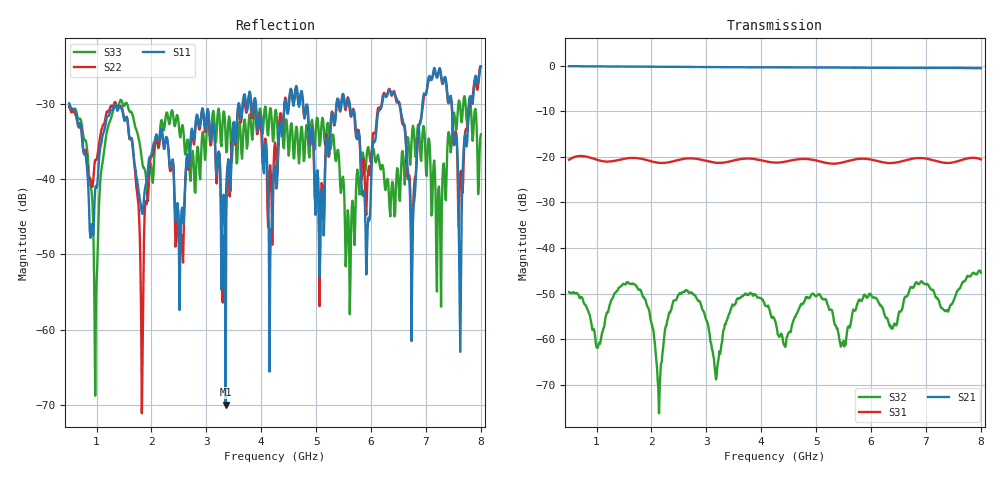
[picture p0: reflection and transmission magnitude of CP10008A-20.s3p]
! Amtery
! Email: info@amtery.com
! Phone: 886-2-2883-7839
! Model Number: CP10008A-20
! 3-port S-parameter measurement data for Directional Coupler
! Frequency Range: 0.5 GHz to 8 GHz
! Port 1: Input
! Port 2: Output
! Port 3: Coupled
# Hz S db R 50
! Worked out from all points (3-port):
!   601 points, 500 MHz to 8 GHz, reference 50 ohm
!   strongest paths, dB at 500 MHz, 2.375 GHz, 4.25 GHz, 6.125 GHz, 8 GHz:
!     S21: -0.1, -0.3, -0.4, -0.5, -0.6
!     S31: -20.6, -21.0, -21.3, -21.0, -20.6
!     S32: -49.7, -52.6, -55.9, -51.6, -45.4
!   lowest |S11| = -70.0 dB at 3.35 GHz (marker M1), VSWR 1.00, Z = 50 - j0.022 ohm
!   |S11| at or under -10 dB: start of sweep to end of sweep
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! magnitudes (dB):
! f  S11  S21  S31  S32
! 500 MHz  -29.9  -0.1  -20.6  -49.7
! 987.5 MHz  -40.9  -0.2  -20.6  -61.1
! 1.325 GHz  -30.2  -0.2  -20.9  -49.9
! 1.825 GHz  -44.5  -0.2  -20.5  -50.1
! 3.35 GHz  -70.0  -0.4  -21.2  -56.7
! 4.25 GHz  -38.2  -0.4  -21.3  -55.9
! 6.75 GHz  -50.9  -0.5  -20.4  -48.6
! 7.25 GHz  -25.2  -0.5  -21.1  -52.3
! 7.625 GHz  -63.0  -0.5  -20.8  -48.7
! 8 GHz  -25.0  -0.6  -20.6  -45.4
